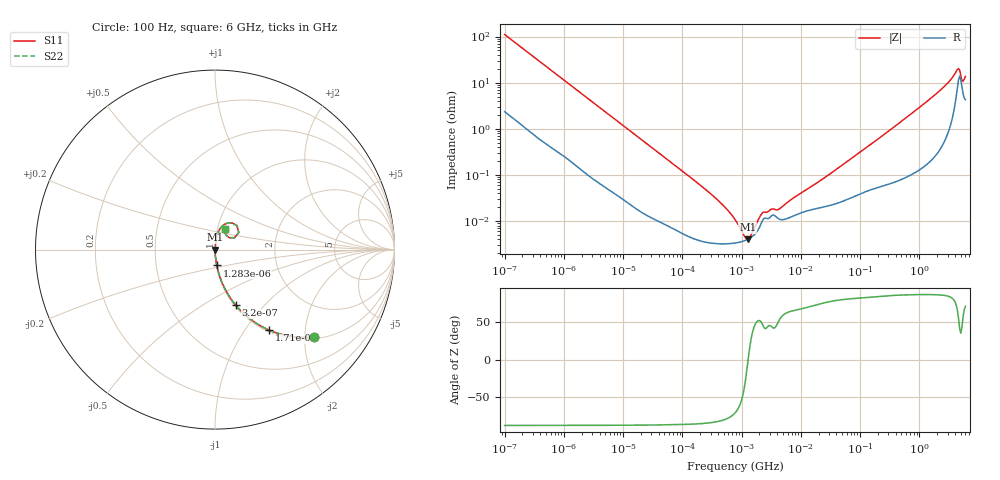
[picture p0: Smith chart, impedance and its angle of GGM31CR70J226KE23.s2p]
!Murata Part Number: GGM31CR70J226KE23
!These Parameters are Measured in Series Mode Connection
!Data Generated on Jun 19, 2026
!  o--ll--o
!Port1  Port2
!  o------o
!Operation Temp=25[degC], DC Bias Voltage=0[V]
!Freq. Start=100[Hz] Stop=6[GHz] 401[Steps]
# Hz S RI R 50
!Freq.(Hz) S11(Real) S11(Imag) S21(Real) S21(Imag) S12(Real) S12(Imag) S22(Real) S22(Imag)
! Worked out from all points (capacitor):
!   401 points, 100 Hz to 6 GHz, reference 50 ohm
!   read as one part in series: C = 14.3 uF near 109 Hz
!   lowest |Z| = 4.04 mohm at 1.268 MHz (marker M1)
!   series resonance near 1.291 MHz, so ESL is about 1.1 nH
!   S11 on the Smith chart (normalised r, x): 100 Hz: 1.05, -2.22; 171 Hz: 1.03, -1.31; 320 Hz: 1.01, -0.70; 1.283 kHz: 1.00, -0.18; 6 GHz: 1.09, +0.26
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100  0.5514 -0.4869  0.4486 0.4869  0.4486 0.4869  0.5514 -0.4869
171  0.3034 -0.4493  0.6966 0.4493  0.6966 0.4493  0.3034 -0.4493
320  0.1153 -0.3093  0.8847 0.3093  0.8847 0.3093  0.1153 -0.3093
1283  0.0099 -0.0885  0.9901 0.0885  0.9901 0.0885  0.0099 -0.0885
2008  0.00455 -0.0573  0.9954 0.0573  0.9954 0.0573  0.00455 -0.0573
40335  0.000107 -0.00299  0.9999 0.00299  0.9999 0.00299  0.000107 -0.00299
316350  3.33e-05 -0.000369  1 0.000369  1 0.000369  3.33e-05 -0.000369
517687  3.21e-05 -0.000202  1 0.000202  1 0.000202  3.21e-05 -0.000202
774597  3.35e-05 -0.000104  1 0.000104  1 0.000104  3.35e-05 -0.000104
885955  3.45e-05 -7.51e-05  1 7.51e-05  1 7.51e-05  3.45e-05 -7.51e-05
1267578  4.02e-05 -3.6e-06  1 3.6e-06  1 3.6e-06  4.02e-05 -3.6e-06
1734173  5.46e-05 6.21e-05  0.9999 -6.21e-05  0.9999 -6.21e-05  5.46e-05 6.21e-05
2372521  0.000114 0.000109  0.9999 -0.000109  0.9999 -0.000109  0.000114 0.000109
4246196  0.000112 0.000142  0.9999 -0.000142  0.9999 -0.000142  0.000112 0.000142
1.555665e7  0.000178 0.000549  0.9998 -0.000549  0.9998 -0.000549  0.000178 0.000549
3.124326e8  0.000722 0.00917  0.9993 -0.00917  0.9993 -0.00917  0.000722 0.00917
2.048624e9  0.00675 0.0608  0.9933 -0.0608  0.9933 -0.0608  0.00675 0.0608
3.352442e9  0.024 0.1099  0.976 -0.1099  0.976 -0.1099  0.024 0.1099
4.193612e9  0.0711 0.1485  0.9289 -0.1485  0.9289 -0.1485  0.0711 0.1485
4.586474e9  0.123 0.1324  0.877 -0.1324  0.877 -0.1324  0.123 0.1324
5.486059e9  0.0619 0.0805  0.9381 -0.0805  0.9381 -0.0805  0.0619 0.0805
6e9  0.0558 0.1174  0.9442 -0.1174  0.9442 -0.1174  0.0558 0.1174
